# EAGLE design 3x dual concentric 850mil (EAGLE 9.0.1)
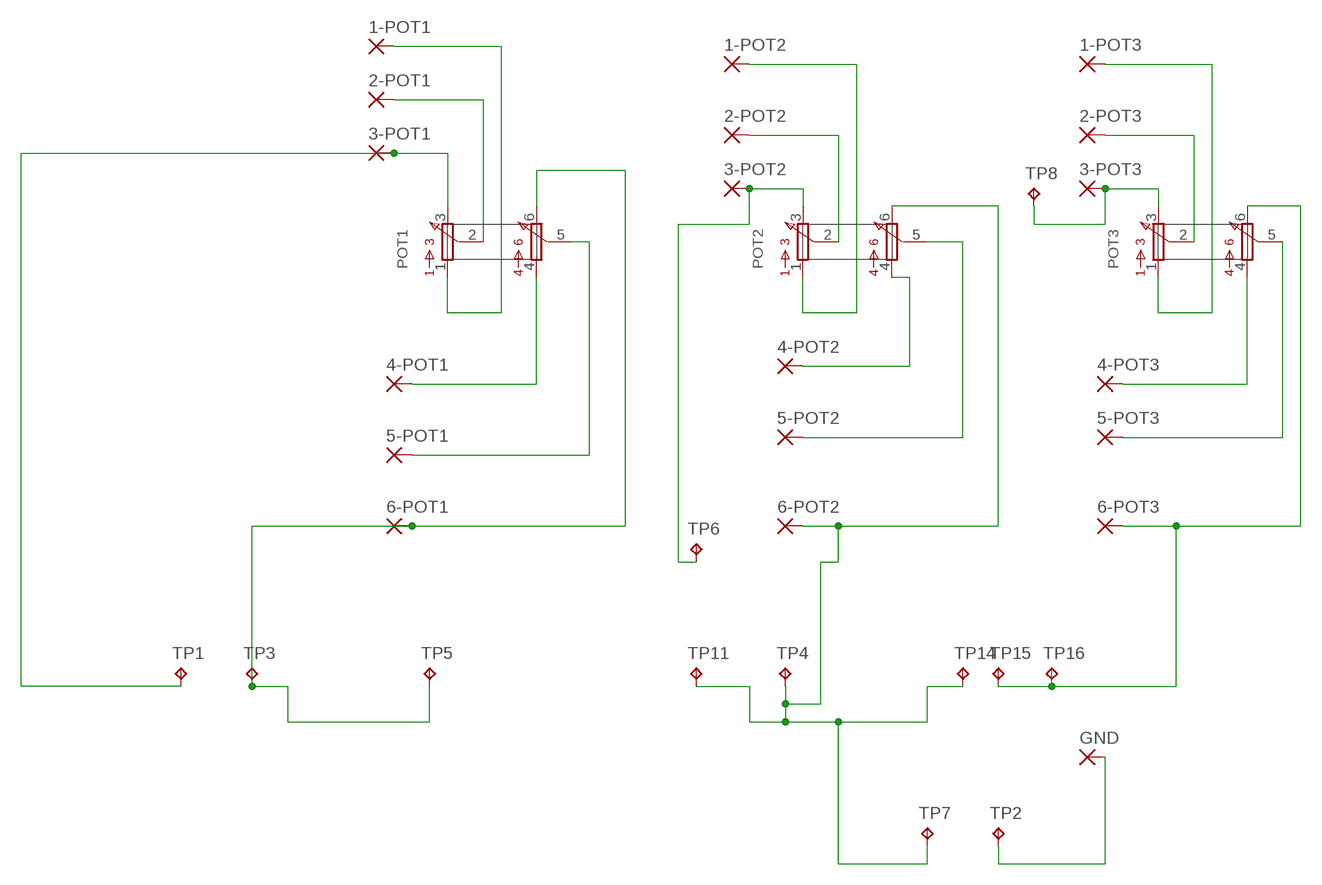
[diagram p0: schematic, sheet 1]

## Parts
1-POT1  WIREPAD2,54/0,9  [2,54/0,9]
1-POT2  WIREPAD2,54/0,9  [2,54/0,9]
1-POT3  WIREPAD2,54/0,9  [2,54/0,9]
2-POT1  WIREPAD2,54/0,9  [2,54/0,9]
2-POT2  WIREPAD2,54/0,9  [2,54/0,9]
2-POT3  WIREPAD2,54/0,9  [2,54/0,9]
3-POT1  WIREPAD2,54/0,9  [2,54/0,9]
3-POT2  WIREPAD2,54/0,9  [2,54/0,9]
3-POT3  WIREPAD2,54/0,9  [2,54/0,9]
4-POT1  WIREPAD2,54/0,9  [2,54/0,9]
4-POT2  WIREPAD2,54/0,9  [2,54/0,9]
4-POT3  WIREPAD2,54/0,9  [2,54/0,9]
5-POT1  WIREPAD2,54/0,9  [2,54/0,9]
5-POT2  WIREPAD2,54/0,9  [2,54/0,9]
5-POT3  WIREPAD2,54/0,9  [2,54/0,9]
6-POT1  WIREPAD2,54/0,9  [2,54/0,9]
6-POT2  WIREPAD2,54/0,9  [2,54/0,9]
6-POT3  WIREPAD2,54/0,9  [2,54/0,9]
GND  WIREPAD2,54/0,9  [2,54/0,9]
POT1  DUALCONCENTRIC  [DUALCONCENTRIC]
POT2  DUALCONCENTRIC  [DUALCONCENTRIC]
POT3  DUALCONCENTRIC  [DUALCONCENTRIC]
TP1  TPPAD1-13  [P1-13]
TP2  TPPAD1-13  [P1-13]
TP3  TPPAD1-13  [P1-13]
TP4  TPPAD1-13  [P1-13]
TP5  TPPAD1-13  [P1-13]
TP6  TPPAD1-13  [P1-13]
TP7  TPPAD1-13  [P1-13]
TP8  TPPAD1-13  [P1-13]
TP11  TPPAD1-13  [P1-13]
TP14  TPPAD1-13  [P1-13]
TP15  TPPAD1-13  [P1-13]
TP16  TPPAD1-13  [P1-13]

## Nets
N$1: 6-POT3.1(P) POT3.6 TP15.TP TP16.TP
N$2: GND.1(P) TP2.TP
N$3: 3-POT3.1(P) POT3.3 TP8.TP
N$4: 2-POT1.1(P) POT1.2
N$5: 2-POT2.1(P) POT2.2
N$6: 2-POT3.1(P) POT3.2
N$7: 3-POT2.1(P) POT2.3 TP6.TP
N$8: 1-POT2.1(P) POT2.1
N$9: 6-POT1.1(P) POT1.6 TP3.TP TP5.TP
N$10: 4-POT1.1(P) POT1.4
N$11: 4-POT2.1(P) POT2.4
N$12: 4-POT3.1(P) POT3.4
N$13: 5-POT3.1(P) POT3.5
N$14: 5-POT1.1(P) POT1.5
N$15: 5-POT2.1(P) POT2.5
N$17: 3-POT1.1(P) POT1.3 TP1.TP
N$19: 1-POT1.1(P) POT1.1
N$21: 6-POT2.1(P) POT2.6 TP4.TP TP7.TP TP11.TP TP14.TP
N$23: 1-POT3.1(P) POT3.1

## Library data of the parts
1-POT1-1-POT3 2-POT1-2-POT3 3-POT1-3-POT3 4-POT1-4-POT3 5-POT1-5-POT3 6-POT1-6-POT3 GND = wirepad-NONAMES:WIREPAD: Wire PAD connect wire on PCB
POT1-POT3 = clonepots:DUALCONCENTRIC: Dual Concentric Pot Alps Clone.
TP1-TP8 TP11 TP14-TP16 = testpad-CL:TP: Test pad NO NAME

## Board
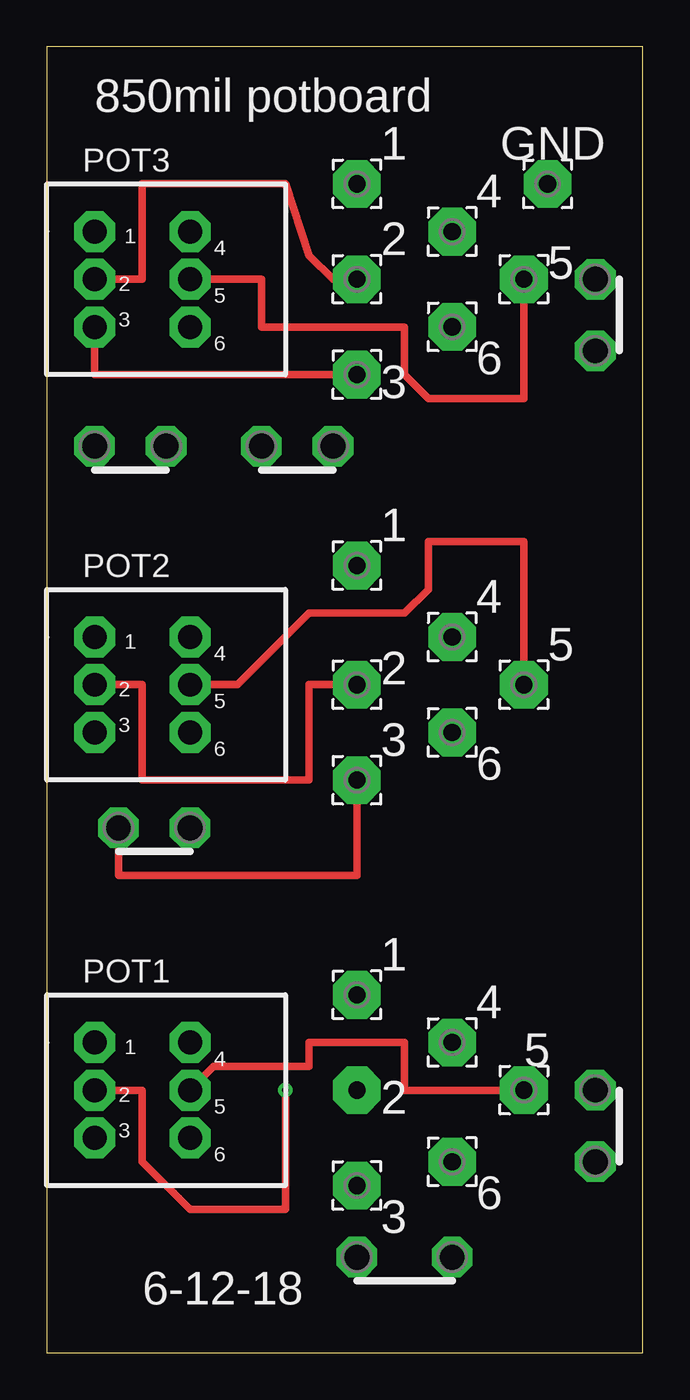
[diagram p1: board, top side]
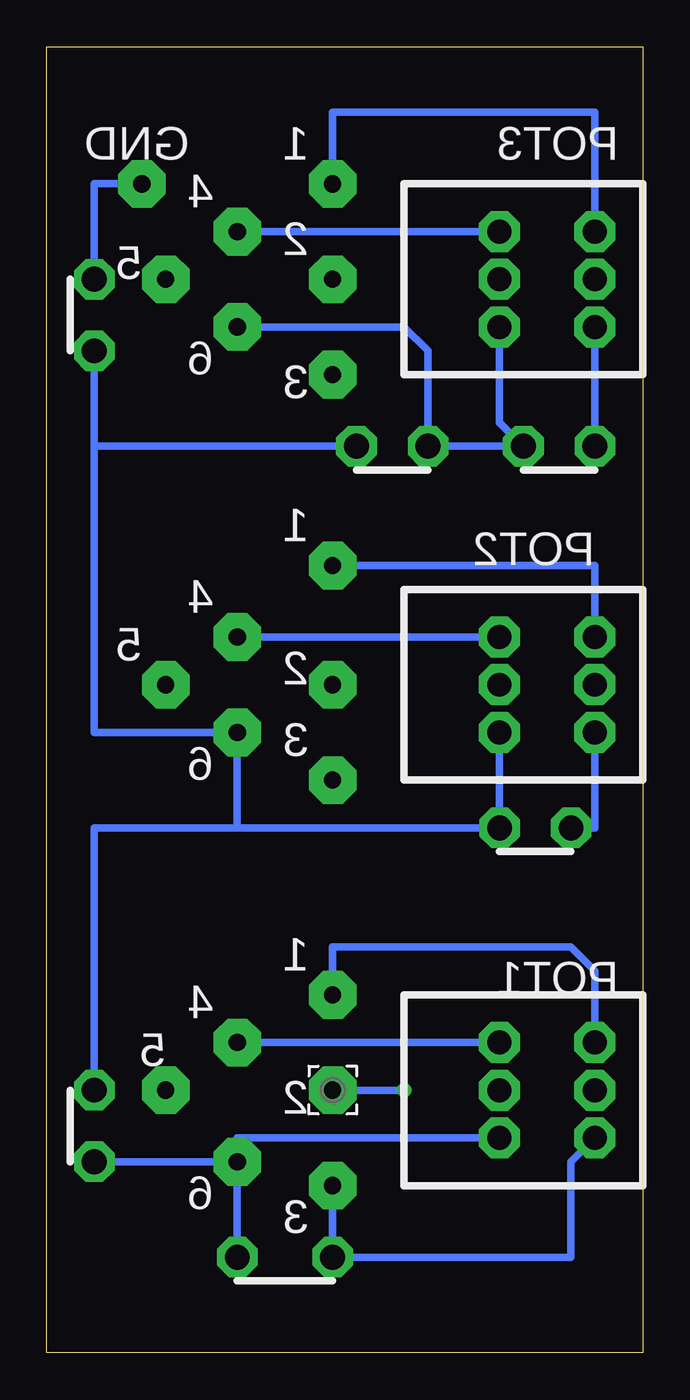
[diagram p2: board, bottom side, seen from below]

Size 31.73 x 69.52 mm. Coordinates in mm from the lower left corner, seen from the top.
Outline: 0,0 31.73,0 31.73,69.52 0,69.52 0,0
Copper layers (1*16): Top 0.035mm / dielectric 1.5mm / Bottom 0.035mm
Design rules "default": minimum track width 6mil, minimum drill 0.35mm, track to track 6mil, track to pad 6mil, pad to pad 6mil, via to via 6mil, smd to smd 6mil, copper to edge 40mil, drill to drill 6mil, minimum pad ring 10mil, minimum via ring 8mil, stop-mask expansion 4mil, vias tented up to drill 0mil, thermal gap 10mil

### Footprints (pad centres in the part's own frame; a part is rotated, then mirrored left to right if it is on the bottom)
2,54/0,9 = drill 0.914 pad 2.54 octagon: 1 0,0
DUALCONCENTRIC = drill 1.27 pad 2.184 octagon: 1 -8.89,2.54; 2 -8.89,0; 3 -8.89,-2.54; 4 -3.81,2.54; 5 -3.81,0; 6 -3.81,-2.54
P1-13 = drill 1.321 pad 2.159 octagon: TP 0,0

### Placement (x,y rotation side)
1-POT1  16.51,19.05 0 top
1-POT2  16.51,41.91 0 top
1-POT3  16.51,62.23 0 top
2-POT1  16.51,13.97 0 bottom
2-POT2  16.51,35.56 0 top
2-POT3  16.51,57.15 0 top
3-POT1  16.51,8.89 0 top
3-POT2  16.51,30.48 0 top
3-POT3  16.51,52.07 0 top
4-POT1  21.59,16.51 0 top
4-POT2  21.59,38.1 0 top
4-POT3  21.59,59.69 0 top
5-POT1  25.4,13.97 0 top
5-POT2  25.4,35.56 0 top
5-POT3  25.4,57.15 0 top
6-POT1  21.59,10.16 0 top
6-POT2  21.59,33.02 0 top
6-POT3  21.59,54.61 0 top
GND  26.67,62.23 0 top
POT1  11.43,13.97 0 top
POT2  11.43,35.56 0 top
POT3  11.43,57.15 0 top
TP1  16.51,5.08 0 top
TP2  29.21,57.15 0 top
TP3  21.59,5.08 0 top
TP4  7.62,27.94 0 top
TP5  29.21,10.16 0 top
TP6  3.81,27.94 0 top
TP7  29.21,53.34 0 top
TP8  2.54,48.26 0 top
TP11  15.24,48.26 0 top
TP14  29.21,13.97 0 top
TP15  6.35,48.26 0 top
TP16  11.43,48.26 0 top

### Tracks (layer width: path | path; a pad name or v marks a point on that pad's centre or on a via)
N$1
  Bottom 0.406: POT3.6 7.62,49.53 TP15.TP TP16.TP 11.43,53.34 12.7,54.61 6-POT3.1
N$2
  Bottom 0.406: TP2.TP 29.21,62.23 GND.1
N$3
  Top 0.406: 3-POT3.1 2.54,52.07 POT3.3
  Bottom 0.406: TP8.TP POT3.3
N$4  (via drill 0.35)
  Top 0.406: POT1.2 5.08,13.97 5.08,10.16 7.62,7.62 12.7,7.62 v12.7,13.97
  Bottom 0.406: v12.7,13.97 2-POT1.1
N$5
  Top 0.406: POT2.2 5.08,35.56 5.08,30.48 13.97,30.48 13.97,35.56 2-POT2.1
N$6
  Top 0.406: POT3.2 5.08,57.15 5.08,62.23 12.7,62.23 13.97,58.42 15.24,57.15 2-POT3.1
N$7
  Top 0.406: TP6.TP 3.81,25.4 16.51,25.4 3-POT2.1
  Bottom 0.406: POT2.3 2.54,27.94 TP6.TP
N$8
  Bottom 0.406: POT2.1 2.54,41.91 1-POT2.1
N$9
  Bottom 0.406: POT1.6 21.59,11.43 6-POT1.1 | TP3.TP 6-POT1.1 | 6-POT1.1 TP5.TP
N$10
  Bottom 0.406: POT1.4 4-POT1.1
N$11
  Bottom 0.406: POT2.4 4-POT2.1
N$12
  Bottom 0.406: POT3.4 4-POT3.1
N$13
  Top 0.406: POT3.5 11.43,57.15 11.43,54.61 19.05,54.61 19.05,52.07 20.32,50.8 25.4,50.8 5-POT3.1
N$14
  Top 0.406: POT1.5 8.89,15.24 13.97,15.24 13.97,16.51 19.05,16.51 19.05,13.97 5-POT1.1
N$15
  Top 0.406: POT2.5 10.16,35.56 13.97,39.37 19.05,39.37 20.32,40.64 20.32,43.18 25.4,43.18 5-POT2.1
N$17
  Bottom 0.406: POT1.3 3.81,10.16 3.81,5.08 TP1.TP 3-POT1.1
N$19
  Bottom 0.406: POT1.1 2.54,20.32 3.81,21.59 16.51,21.59 1-POT1.1
N$21
  Bottom 0.406: 21.59,27.94 TP4.TP POT2.6 | 21.59,27.94 29.21,27.94 TP14.TP | 21.59,27.94 6-POT2.1 29.21,33.02 29.21,48.26 | 29.21,48.26 TP11.TP | TP7.TP 29.21,48.26
N$23
  Bottom 0.406: POT3.1 2.54,66.04 16.51,66.04 1-POT3.1

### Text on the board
tNames: 850mil potboard | 1 | GND | 4 | 2 | 5 | 6 | 3 | 1 | 4 | 5 | 2 | 3 | 6 | 1 | 4 | 5 | 2 | 2 | 6 | 3 | 6-12-18
bNames: POT3 | 1 | GND | 4 | 2 | 5 | 6 | 3 | 1 | POT2 | 4 | 5 | 2 | 3 | 6 | 1 | POT1 | 4 | 5 | 2 | 6 | 3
